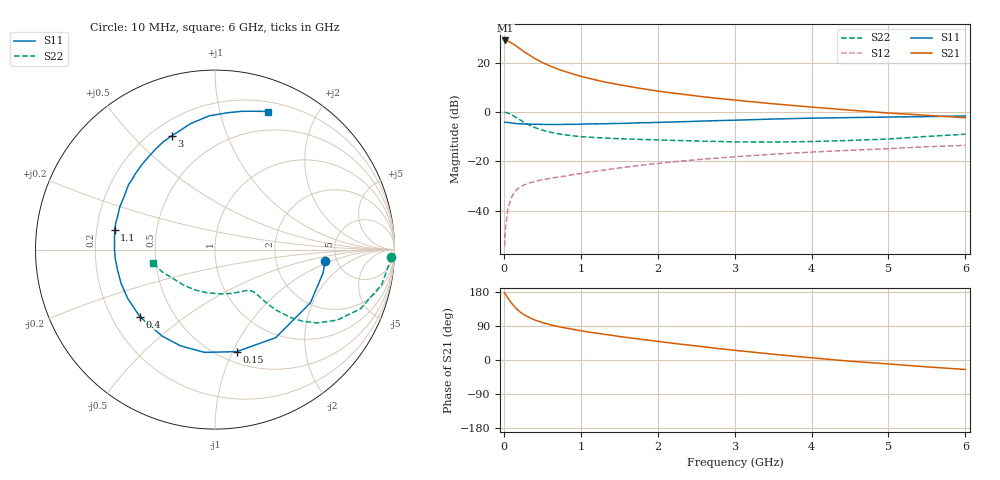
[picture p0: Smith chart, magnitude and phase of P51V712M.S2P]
! SIEMENS Small Signal Semiconductors
! BFP183
! Si NPN RF Bipolar Junction Transistor in SOT143
! VCE = 1.75 V  IC = 12 mA
! Common Emitter S-Parameters:  March  1996
# GHz  S  MA  R  50
!  f  S11  S21  S12  S22
! GHz  MAG  ANG  MAG  ANG  MAG  ANG  MAG  ANG
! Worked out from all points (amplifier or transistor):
!   36 points, 10 MHz to 6 GHz, reference 50 ohm
!   highest |S21| = 28.9 dB at 20 MHz (marker M1)
!   |S21| within 3 dB of that: start of sweep to 193.4 MHz
!   unconditionally stable (mu >= 1): 984.4 MHz to 5.624 GHz
!   at 250 MHz: K = 0.38, MSG = 27.2 dB, |S12| = -29.8 dB
!   at 1.4 GHz: K = 1.11, MAG = 15.3 dB, |S12| = -23.1 dB
!   at 6 GHz: K = 0.95, MSG = 5.6 dB, |S12| = -13.6 dB
!   S11 on the Smith chart (normalised r, x): 10 MHz: 4.03, -0.81; 150 MHz: 0.60, -1.04; 400 MHz: 0.32, -0.35; 1.1 GHz: 0.28, +0.09; 3 GHz: 0.28, +0.65; 6 GHz: 0.29, +1.42
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0.01  0.6157 -5.8  27.93 176.9  0.0019 83.7  0.9801 -2.4
0.02  0.6165 -12.0  27.98 173.9  0.0043 85.2  0.9726 -4.8
0.05  0.6087 -29.1  27.35 164.1  0.0104 77.8  0.9494 -11.8
0.1  0.5959 -55.4  24.78 150.0  0.0187 66.6  0.8755 -22.1
0.15  0.5812 -78.0  22.13 138.1  0.025 58.1  0.7859 -30.0
0.2  0.5757 -95.9  19.48 128.6  0.0292 53.0  0.7016 -35.6
0.25  0.5695 -109.7  17.05 121.2  0.0322 48.7  0.6298 -39.3
0.3  0.5648 -121.3  15.14 115.3  0.035 46.9  0.5692 -41.8
0.4  0.5612 -138.3  12.14 105.7  0.0389 43.8  0.4827 -44.6
0.5  0.5574 -150.6  9.981 98.9  0.042 42.6  0.426 -45.8
0.6  0.5561 -160.2  8.552 93.3  0.0448 42.6  0.3879 -46.3
0.7  0.5548 -168.4  7.365 88.6  0.0475 43.4  0.3608 -46.6
0.9  0.5599 179.5  5.851 80.9  0.0536 44.3  0.3266 -47.3
1.1  0.5696 168.9  4.816 73.8  0.0602 45.4  0.3072 -48.7
1.5  0.5827 153.8  3.548 62.1  0.0729 46.4  0.2864 -53.0
1.8  0.6027 143.0  2.953 54.1  0.0833 45.8  0.2751 -57.8
2.2  0.624 131.0  2.403 44.1  0.0969 44.2  0.2645 -65.6
3  0.6778 110.8  1.734 25.7  0.1229 39.1  0.2462 -85.5
3.5  0.7152 100.9  1.458 15.2  0.1386 35.5  0.2445 -100.0
4.5  0.7656 84.8  1.084 -3.2  0.1662 27.5  0.2638 -131.4
5.5  0.8023 73.9  0.852 -18.1  0.1968 20.2  0.3179 -156.5
6  0.8246 68.9  0.762 -25.0  0.2095 15.6  0.3526 -167.4
